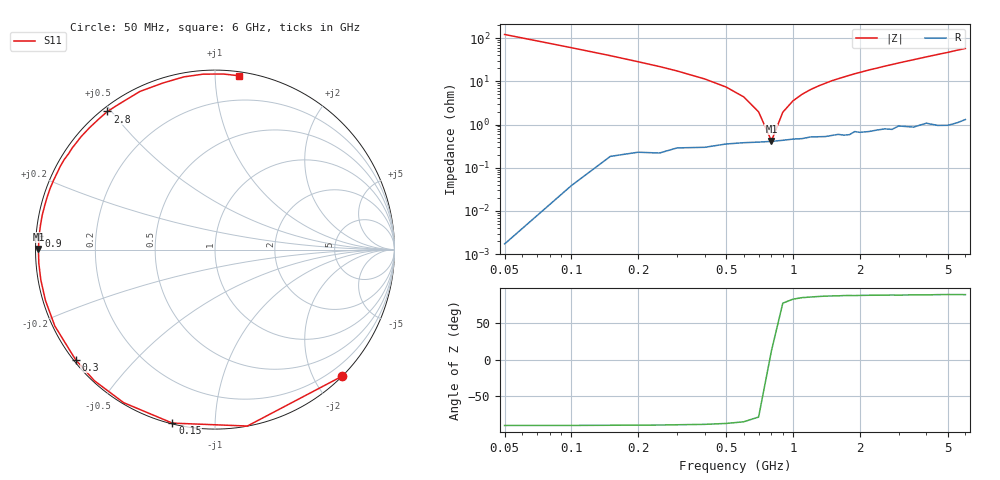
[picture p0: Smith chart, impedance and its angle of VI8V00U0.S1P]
! Infineon Technologies  Discrete & RF Semiconductors
! BB 804
! Si Tuning Diode in SOT23
! VR = 8 V
! S-Parameters:  July  1999
# GHz  S  MA  R  50
!  f  S11
! GHz  MAG  ANG
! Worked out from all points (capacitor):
!   34 points, 50 MHz to 6 GHz, reference 50 ohm
!   read as one part to ground: C = 26.1 pF near 50 MHz
!   lowest |Z| = 416 mohm at 800 MHz (marker M1)
!   series resonance near 795.7 MHz, so ESL is about 1.5 nH
!   S11 on the Smith chart (normalised r, x): 50 MHz: 0.00, -2.43; 150 MHz: 0.00, -0.78; 300 MHz: 0.01, -0.35; 900 MHz: 0.01, +0.04; 2.8 GHz: 0.02, +0.49; 6 GHz: 0.03, +1.15
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0.05  1 -44.8
0.1  0.9994 -79.6
0.15  0.9955 -103.8
0.2  0.9931 -120.8
0.25  0.9927 -132.6
0.3  0.9898 -141.7
0.4  0.9888 -154.5
0.5  0.9862 -163.3
0.6  0.9851 -170.1
0.7  0.9845 -175.6
0.8  0.9839 179.8
0.9  0.9829 175.7
1  0.9819 172.0
1.2  0.98 165.4
1.5  0.9788 156.7
1.6  0.9778 154.2
1.8  0.9786 149.2
2  0.9764 144.5
2.2  0.976 139.9
2.4  0.9747 135.9
2.6  0.974 131.6
2.8  0.9754 127.9
3.5  0.9754 115.4
4  0.9725 107.4
4.5  0.9778 100.2
5  0.9797 93.9
5.5  0.9794 87.3
6  0.9778 82.1
